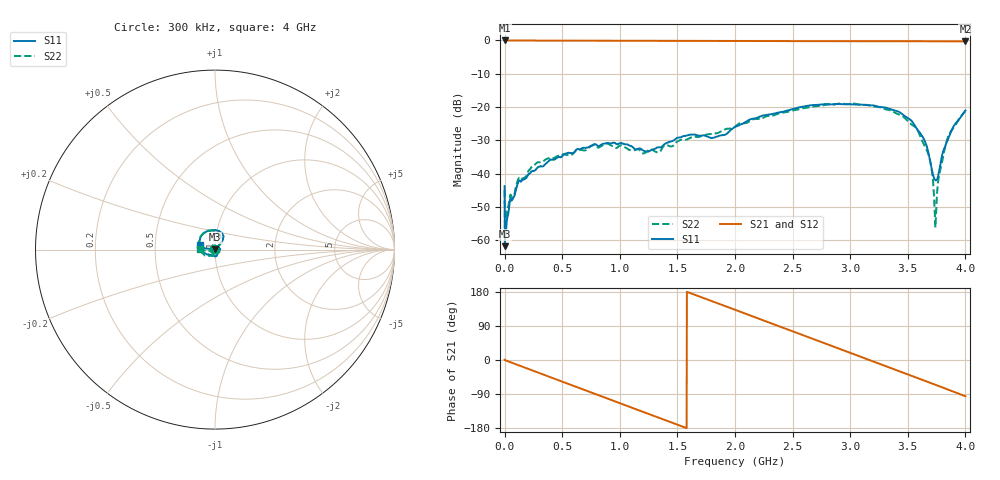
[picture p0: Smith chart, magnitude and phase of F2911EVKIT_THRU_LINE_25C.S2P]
! Integrated Device Technology
! Corporate Headquarters
! 6024 Silver Creek Valley Road
! San Jose, CA 95138  USA
! Phone:  1-408-284-8200
! Toll Free:  1-800-223-1366
! Webpage:  http://www.idt.com/
! Timing and RF Division
! 515 Groton Road, Suite 102
! Westford, MA 01886-6024
! Description: F2911 EVKIT Thru Line
! Frequency:  300 kHz to 4 GHz
! Ports:  2 RF, 0 DC
!  EVKit RF Connector J4  = Port 1
!  EVKit RF Connector J5  = Port 2
! Data:  The results below were measured on the F2911 EVKit Thru Line from J4 to J5
!  using a calibrated network analyzer. The reference plane is at
!  the SMA coaxial interfaces.
! Misc:
! Date Measured:  2017-08-11
! Date:  2017-09-21  SJ
! Note:
!  Integrated Device Technology supplies this data as a sample
!	of measured data. Data was taken at 25 degrees C.
!  Integrated Device Technology reserves the right to change
! 	this data at anytime.
!PortZ  Port1:75+j0  Port2:75+j0
# Hz S dB R 75
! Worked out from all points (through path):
!   1601 points, 300 kHz to 4 GHz, reference 75 ohm
!   highest |S21| = -0.01 dB at 2.8 MHz (marker M1); lowest = -0.3 dB at 4 GHz (marker M2)
!   group delay of S21, straight-line fit = 316 ps
!   lowest |S11| = -61.7 dB at 2.8 MHz (marker M3), VSWR 1.00, Z = 75 + j0.117 ohm
!   |S11| at or under -10 dB: start of sweep to end of sweep
!   |S22| runs from -58.3 to -18.9 dB; largest |S21 - S12| = 0.0017
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300000  -43.72 128.7  -0.01 0.6  -0.01 0.6  -44.84 120.0
2799813  -61.72 72.3  -0.01 -0.3  -0.01 -0.3  -58.31 30.5
2.279831e7  -53.27 42.2  -0.02 -2.6  -0.02 -2.7  -50.75 33.2
5.029625e7  -47.57 40.5  -0.02 -5.8  -0.02 -5.8  -46.30 34.0
1.177912e8  -42.58 51.2  -0.03 -13.5  -0.03 -13.6  -41.67 43.8
2.752794e8  -38.55 47.1  -0.04 -31.5  -0.04 -31.5  -36.86 36.0
6.677499e8  -32.39 16.2  -0.07 -76.2  -0.07 -76.2  -32.84 -5.9
9.852261e8  -31.09 1.9  -0.08 -112.2  -0.08 -112.3  -31.94 -37.9
1.3352e9  -32.04 -49.8  -0.09 -151.9  -0.09 -152.0  -33.63 -84.1
1.662675e9  -28.35 -84.1  -0.12 170.8  -0.13 170.8  -28.90 -110.1
1.812664e9  -29.20 -108.3  -0.14 153.7  -0.14 153.7  -27.91 -120.2
2.00015e9  -25.96 -147.4  -0.14 132.4  -0.14 132.4  -25.90 -138.1
2.335125e9  -22.00 175.5  -0.18 94.4  -0.18 94.4  -22.49 -169.5
2.6676e9  -19.40 138.3  -0.22 56.8  -0.23 56.7  -19.92 151.9
3.010074e9  -19.16 98.9  -0.25 18.0  -0.25 18.0  -18.96 112.2
3.33505e9  -20.46 63.4  -0.25 -18.8  -0.25 -18.9  -20.87 76.0
3.590031e9  -27.05 46.2  -0.24 -48.0  -0.25 -48.1  -27.32 50.8
3.687523e9  -35.00 50.9  -0.24 -59.3  -0.25 -59.4  -35.13 38.5
3.74002e9  -41.93 84.0  -0.25 -65.4  -0.25 -65.4  -56.11 140.5
3.780016e9  -37.65 156.6  -0.25 -70.0  -0.26 -70.1  -39.17 -152.8
3.842512e9  -30.18 172.2  -0.25 -77.3  -0.26 -77.3  -29.60 -166.8
4e9  -21.03 163.8  -0.30 -95.7  -0.30 -95.7  -21.30 176.6
